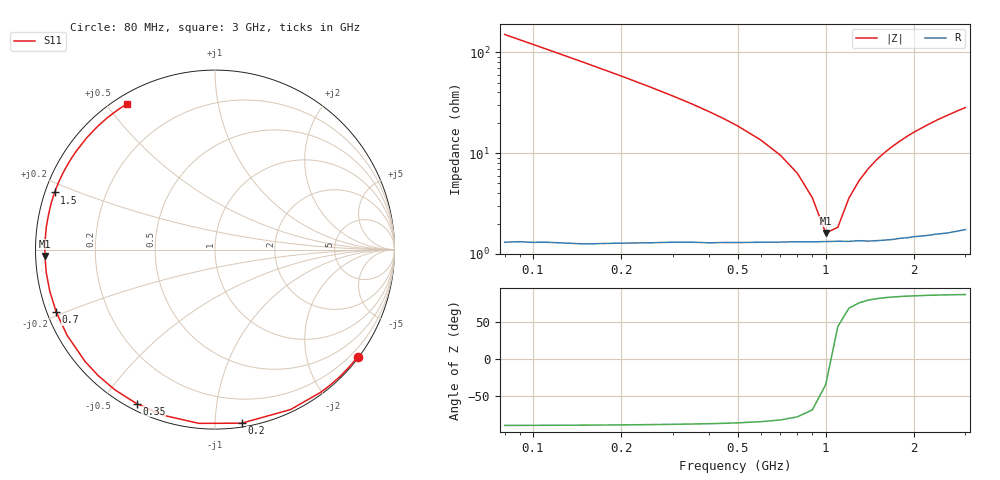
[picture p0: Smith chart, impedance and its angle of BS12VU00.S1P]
! SIEMENS Small Signal Semiconductors
! BB640
! Si Tuning Diode in SOD323
! VR = 12 V
! S-Parameters:  July  1993
# GHz  S  MA  R  50
!  f  S11
! GHz  MAG  ANG
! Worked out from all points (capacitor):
!   33 points, 80 MHz to 3 GHz, reference 50 ohm
!   read as one part to ground: C = 13.2 pF near 80 MHz
!   lowest |Z| = 1.61 ohm at 1 GHz (marker M1)
!   series resonance near 1.042 GHz, so ESL is about 1.8 nH
!   S11 on the Smith chart (normalised r, x): 80 MHz: 0.03, -3.01; 200 MHz: 0.03, -1.16; 350 MHz: 0.03, -0.61; 700 MHz: 0.03, -0.19; 1.5 GHz: 0.03, +0.17; 3 GHz: 0.03, +0.57
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0.08  0.9948 -36.8
0.1  0.9923 -45.3
0.11  0.9909 -49.4
0.12  0.9896 -53.4
0.15  0.9857 -64.7
0.2  0.9785 -81.3
0.25  0.9722 -95.3
0.3  0.9667 -107.1
0.35  0.9627 -117.0
0.4  0.96 -125.5
0.45  0.9573 -132.8
0.5  0.9554 -139.2
0.6  0.9524 -149.9
0.7  0.9506 -158.6
0.8  0.9493 -165.9
0.9  0.9488 -172.3
1  0.9483 -177.9
1.2  0.9483 172.4
1.4  0.9487 164.2
1.5  0.9487 160.4
1.6  0.9486 156.9
1.8  0.9479 150.4
2  0.9476 144.4
2.2  0.948 139.0
2.4  0.948 133.9
2.6  0.9486 129.4
2.8  0.9485 125.0
3  0.9485 121.0
